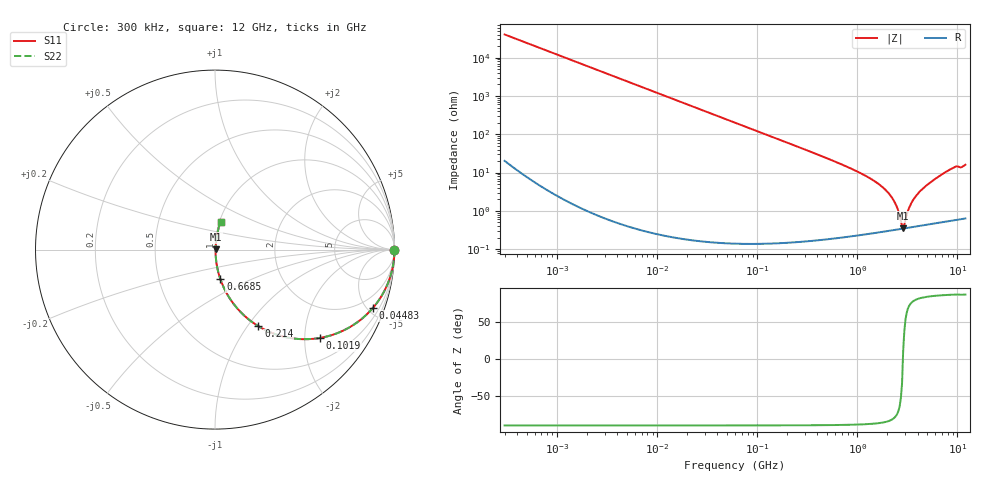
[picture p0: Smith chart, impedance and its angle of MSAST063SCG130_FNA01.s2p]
! MSAST063SCG130_FNA01  S-PARAMETER MODEL  ( Standard Model )
! Model Generated by TAIYO YUDEN Corporation (http://www.ty-top.com)
! Version 1.0
! TAIYO YUDEN Control No. 241122
! Copyright(c) 2024 TAIYO YUDEN CO.,LTD. All Rights Reserved.
! Product Description (link to TY-COMPAS)
! https://ds.yuden.co.jp/TYCOMPAS/or/detail?pn=MSAST063SCG130JFNA01&u=M
! Products Name : Multilayer Ceramic Capacitors
! Characteristics :
!  Capacitance : 13 [pF] , Rated Voltage : 25 [V] , TCC : CG / C0G
!  Case Size : 0.6 x 0.3 / 0.024 x 0.012 [mm/inch] , Thickness : 0.3 / 0.012 [mm/inch]
!  (Conditions: Temperature = 25 [degC] , DC Bias Voltage = 0 [V])
! External Node Assignments :
!  1  o---| |---o  2
! GND o---------o GND
! Frequency Range : 0.3MHz  -  12000MHz  [ 401 STEP ]
# MHZ S RI R 50
! Freq[MHz].  S11 Real  S11 Imag  S21 Real  S21 Imag  S12 Real  S12 Imag  S22 Real  S22 Imag
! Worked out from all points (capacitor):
!   401 points, 300 kHz to 12 GHz, reference 50 ohm
!   read as one part in series: C = 13.1 pF near 316.3 kHz
!   lowest |Z| = 352 mohm at 2.87 GHz (marker M1)
!   series resonance near 2.852 GHz, so ESL is about 240 pH
!   S11 on the Smith chart (normalised r, x): 300 kHz: open; 44.83 MHz: 1.00, -5.41; 101.9 MHz: 1.00, -2.38; 214 MHz: 1.00, -1.13; 668.5 MHz: 1.00, -0.34; 12 GHz: 1.01, +0.32
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0.3  1 -0.00247  7.37e-06 0.00247  7.37e-06 0.00247  1 -0.00247
1.769972  0.9998 -0.0146  0.000216 0.0146  0.000216 0.0146  0.9998 -0.0146
10.44266  0.9926 -0.0855  0.00738 0.0855  0.00738 0.0855  0.9926 -0.0855
25.03118  0.959 -0.198  0.041 0.198  0.041 0.198  0.959 -0.198
44.83267  0.8795 -0.3253  0.1205 0.3253  0.1205 0.3253  0.8795 -0.3253
60  0.8029 -0.3975  0.1971 0.3975  0.1971 0.3975  0.8029 -0.3975
101.9188  0.5851 -0.4921  0.4149 0.4921  0.4149 0.4921  0.5851 -0.4921
213.9924  0.2415 -0.4267  0.7585 0.4267  0.7585 0.4267  0.2415 -0.4267
353.9943  0.1033 -0.3019  0.8967 0.3019  0.8967 0.3019  0.1033 -0.3019
668.5285  0.0304 -0.1659  0.9696 0.1659  0.9696 0.1659  0.0304 -0.1659
1403.667  0.00683 -0.0651  0.9932 0.0651  0.9932 0.0651  0.00683 -0.0651
2088.533  0.00375 -0.0271  0.9963 0.0271  0.9963 0.0271  0.00375 -0.0271
2384.334  0.00343 -0.0156  0.9966 0.0156  0.9966 0.0156  0.00343 -0.0156
2514.07  0.00338 -0.0111  0.9966 0.0111  0.9966 0.0111  0.00338 -0.0111
2722.03  0.00338 -0.00438  0.9966 0.00438  0.9966 0.00438  0.00338 -0.00438
2870.14  0.00344 0.000703  0.9966 -0.000703  0.9966 -0.000703  0.00344 0.000703
2947.191  0.00348 0.00272  0.9965 -0.00272  0.9965 -0.00272  0.00348 0.00272
3454.93  0.00395 0.0153  0.996 -0.0153  0.996 -0.0153  0.00395 0.0153
4385.161  0.00534 0.0348  0.9947 -0.0348  0.9947 -0.0348  0.00534 0.0348
8064.993  0.0177 0.1101  0.9823 -0.1101  0.9823 -0.1101  0.0177 0.1101
9454.42  0.0247 0.1363  0.9753 -0.1363  0.9753 -0.1363  0.0247 0.1363
12000  0.0309 0.1545  0.9691 -0.1545  0.9691 -0.1545  0.0309 0.1545
